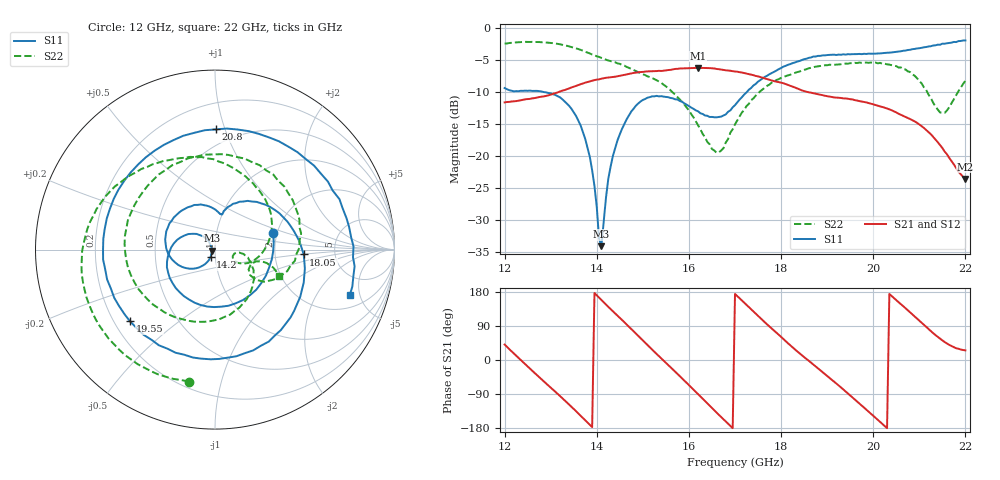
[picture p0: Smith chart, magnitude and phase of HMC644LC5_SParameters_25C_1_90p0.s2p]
!Analog Devices Inc..
!GaAs MMIC 5-BIT DIGITAL PHASE SHIFTER, 15 -8.5 GHz
!Filename: HMC644LC5_sparm_25C_1_0.s2p
!  :25C = 25degC
!  :_1_ = Sn1
!  :_90p0  = 90deg
!Device type:
!2 Port Calibration to sma connectors
!Phase Shifter:  0.000
!	50 Ohm System, Control Voltage = 0/-3V
!Freq	S11	S11	S21	S21	S12	S12	S22	S22
! GHz	Mag dB	Degrees	Mag dB	Degrees	Mag dB	Degrees	Mag dB	Degrees
# GHZ S DB R 50.0
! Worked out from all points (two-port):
!   201 points, 12 GHz to 22 GHz, reference 50 ohm
!   highest |S21| = -6.30 dB at 16.2 GHz (marker M1); lowest = -23.7 dB at 22 GHz (marker M2)
!   |S21| within 3 dB of the highest: 13.47 GHz to 18.28 GHz (4.805 GHz wide, 30.3 % of centre)
!   lowest |S11| = -34.1 dB at 14.1 GHz (marker M3), VSWR 1.04, Z = 48.2 - j0.613 ohm
!   |S11| at or under -10 dB: 12.81 GHz to 17.27 GHz (4.455 GHz wide, 29.6 % of centre)
!   |S22| runs from -19.6 to -2.2 dB; largest |S21 - S12| = 0.0027
!   S11 on the Smith chart (normalised r, x): 12 GHz: 1.90, +0.40; 14.2 GHz: 0.95, -0.08; 18.05 GHz: 2.94, -0.21; 19.55 GHz: 0.26, -0.34; 20.8 GHz: 0.38, +0.93; 22 GHz: 2.92, -4.00
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12  -9.45 16.2  -11.69 40.9  -11.69 40.9  -2.50 -101.2
12.65  -9.89 -90.8  -11.02 -34.1  -11.01 -34.0  -2.26 -143.4
13.2  -10.89 -159.8  -9.99 -94.8  -10.02 -94.7  -2.61 -179.3
13.7  -16.34 144.7  -8.74 -152.9  -8.71 -152.9  -3.62 147.7
13.9  -22.30 128.8  -8.30 -177.1  -8.30 -177.1  -4.22 135.4
14.1  -34.14 -161.1  -7.99 158.5  -8.00 158.7  -4.74 123.5
14.2  -26.57 -121.3  -7.85 146.5  -7.86 146.6  -5.02 117.4
14.65  -14.31 -147.7  -7.32 93.6  -7.31 93.7  -6.16 87.9
15.35  -10.75 146.3  -6.76 10.0  -6.76 10.2  -8.43 36.8
16.2  -13.09 89.0  -6.30 -90.3  -6.30 -90.2  -15.28 -27.2
16.6  -14.02 79.1  -6.47 -138.7  -6.44 -138.6  -19.55 -20.3
17  -12.12 73.3  -6.86 174.4  -6.85 174.5  -15.11 -12.1
17.5  -8.45 41.1  -7.63 116.2  -7.60 116.3  -10.31 -48.9
18.05  -6.11 -3.2  -8.70 55.3  -8.70 55.3  -7.75 -100.8
18.7  -4.53 -59.7  -10.26 -11.8  -10.26 -11.9  -6.20 -163.1
19.15  -4.24 -101.5  -10.92 -57.0  -10.91 -57.0  -5.81 151.2
19.55  -4.16 -139.9  -11.23 -98.8  -11.26 -99.0  -5.60 111.5
19.95  -4.10 179.9  -11.89 -142.1  -11.88 -141.7  -5.46 72.0
20.35  -3.92 137.5  -12.78 174.3  -12.77 174.6  -5.79 32.6
20.8  -3.48 89.7  -14.29 125.8  -14.29 126.0  -6.95 -8.0
21.45  -2.69 26.7  -18.36 56.2  -18.31 56.0  -13.26 -30.6
22  -2.02 -18.8  -23.66 25.5  -23.73 25.5  -8.32 -22.1
